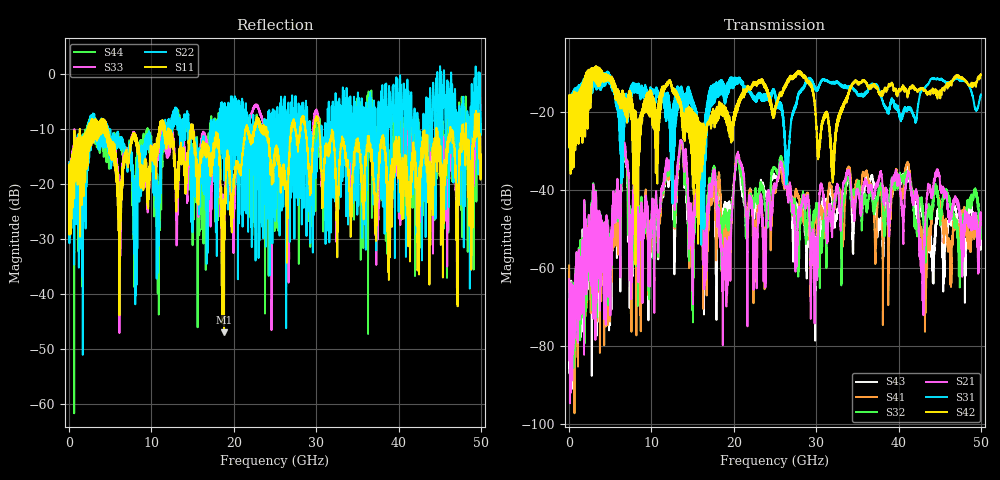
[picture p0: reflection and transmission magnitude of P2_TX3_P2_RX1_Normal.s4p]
!Keysight Technologies,N5225B,MY57041031,A.13.20.10
!Date: Friday, May 31, 2019 11:27:31
!Correction: S11(Full 4 Port(1,2,3,4))
!S12(Full 4 Port(1,2,3,4))
!S13(Full 4 Port(1,2,3,4))
!S14(Full 4 Port(1,2,3,4))
!S21(Full 4 Port(1,2,3,4))
!S22(Full 4 Port(1,2,3,4))
!S23(Full 4 Port(1,2,3,4))
!S24(Full 4 Port(1,2,3,4))
!S31(Full 4 Port(1,2,3,4))
!S32(Full 4 Port(1,2,3,4))
!S33(Full 4 Port(1,2,3,4))
!S34(Full 4 Port(1,2,3,4))
!S41(Full 4 Port(1,2,3,4))
!S42(Full 4 Port(1,2,3,4))
!S43(Full 4 Port(1,2,3,4))
!S44(Full 4 Port(1,2,3,4))
!S4P File: Measurements: <S11,S12,S13,S14>,
!<S21,S22,S23,S24>,
!<S31,S32,S33,S34>,
!<S41,S42,S43,S44>:
# Hz S  dB  R 50.0
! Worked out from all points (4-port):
!   5000 points, 10 MHz to 50 GHz, reference 50 ohm
!   strongest paths, dB at 10 MHz, 12.51 GHz, 25.01 GHz, 37.51 GHz, 50 GHz:
!     S42: -19.4, -14.2, -20.0, -14.4, -10.5
!     S31: -19.5, -43.0, -16.0, -13.6, -15.6
!     S21: -63.0, -32.9, -39.0, -38.1, -47.7
!     S32: -70.6, -34.8, -34.7, -41.8, -48.4
!     S41: -59.4, -35.8, -40.9, -42.4, -49.7
!     S43: -61.1, -38.0, -36.9, -48.8, -51.1
!   lowest |S11| = -47.0 dB at 18.82 GHz (marker M1), VSWR 1.01, Z = 49.6 + j0.0955 ohm
!   |S11| at or under -10 dB: 4.63 GHz to 10.95 GHz (6.318 GHz wide, 81.1 % of centre); 15.04 GHz to 21.46 GHz (6.426 GHz wide, 35.2 % of centre); 30.38 GHz to 44.61 GHz (14.22 GHz wide, 37.9 % of centre)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
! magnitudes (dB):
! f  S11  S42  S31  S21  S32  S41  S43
! 10 MHz  -19.6  -19.4  -19.5  -63.0  -70.6  -59.4  -61.1
! 6.67 GHz  -15.2  -16.1  -20.2  -28.6  -29.5  -29.1  -30.2
! 8.66 GHz  -18.5  -21.3  -14.4  -51.6  -47.7  -63.2  -57.6
! 13.62 GHz  -14.3  -18.4  -14.5  -27.3  -27.6  -28.5  -28.7
! 18.82 GHz  -47.0  -19.6  -13.3  -55.6  -46.1  -47.3  -44.0
! 20.51 GHz  -16.8  -17.2  -11.6  -30.3  -31.3  -30.3  -31.4
! 50 GHz  -15.7  -10.5  -15.6  -47.7  -48.4  -49.7  -51.1
